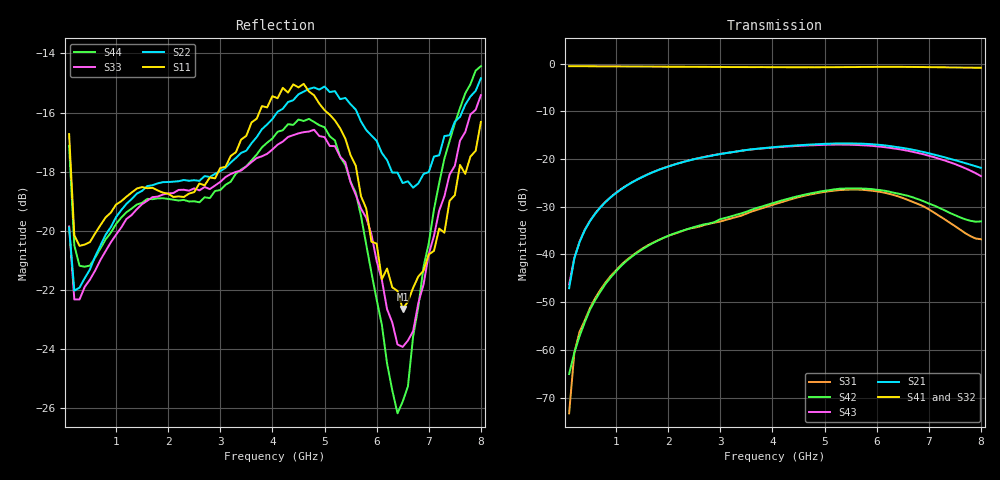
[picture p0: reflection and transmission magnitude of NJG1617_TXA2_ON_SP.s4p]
! Created Wed Nov 12 21:19:47 2008
# hz S ma R 50
! 4 Port Network Data from SP1.SP block
! freq  magS11  angS11  magS12  angS12  magS13  angS13  magS14  angS14
!  magS21  angS21  magS22  angS22  magS23  angS23  magS24  angS24
!  magS31  angS31  magS32  angS32  magS33  angS33  magS34  angS34
!  magS41  angS41  magS42  angS42  magS43  angS43  magS44  angS44
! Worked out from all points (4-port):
!   80 points, 100 MHz to 8 GHz, reference 50 ohm
!   strongest paths, dB at 100 MHz, 2.1 GHz, 4.1 GHz, 6.1 GHz, 8 GHz:
!     S41: -0.6, -0.7, -0.8, -0.7, -0.9
!     S32: -0.5, -0.7, -0.8, -0.7, -1.0
!     S21: -47.1, -21.2, -17.4, -17.1, -21.9
!     S43: -46.3, -21.2, -17.5, -17.5, -23.6
!     S42: -65.0, -35.7, -29.0, -26.6, -33.1
!     S31: -73.3, -35.7, -29.3, -27.0, -36.8
!   lowest |S11| = -22.6 dB at 6.5 GHz (marker M1), VSWR 1.16, Z = 47.3 - j6.64 ohm
!   |S11| at or under -10 dB: start of sweep to end of sweep
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1e8  0.1457 64.7  0.004651 69.8  0.0005039 148.8  0.9386 -8.5
     0.004425 77.5  0.1013 52.7  0.9429 -6.3  0.000954 106.6
     0.0002167 82.8  0.9414 -6.2  0.1017 57.0  0.004587 60.9
     0.9375 -8.4  0.0005592 95.9  0.004852 70.9  0.1391 54.1
2e8  0.09827 48.1  0.009092 80.1  0.0009035 99.5  0.9371 -6.6
     0.009065 79.9  0.07919 35.8  0.9345 -5.3  0.0009284 95.9
     0.0009352 96.7  0.9347 -5.2  0.07652 37.5  0.009224 78.7
     0.9374 -6.5  0.0009347 94.5  0.009199 79.1  0.0944 37.5
5e8  0.0957 39.3  0.02232 79.7  0.00273 102.3  0.9363 -10.2
     0.02234 79.8  0.08603 35.1  0.9348 -9.3  0.002599 102.3
     0.002744 101.9  0.9352 -9.3  0.0827 36.4  0.02252 78.8
     0.9363 -10.1  0.002642 102.8  0.02248 79.1  0.08734 34.5
1.5e9  0.1185 31.8  0.06457 66.2  0.01153 88.4  0.9286 -25.7
       0.06451 66.4  0.1168 32.5  0.9289 -24.6  0.01132 89.6
       0.01149 88.4  0.93 -24.4  0.1109 39.6  0.06491 65.2
       0.9297 -25.5  0.01129 89.8  0.06481 65.4  0.1115 36.3
5e9  0.16 -24.8  0.1442 15.4  0.04524 31.6  0.9143 -82.7
     0.1441 15.4  0.1754 -22.4  0.9127 -79.8  0.04636 30.4
     0.04528 31.8  0.9131 -79.7  0.144 17.5  0.1408 11.2
     0.9152 -82.6  0.04639 30.5  0.1408 11.3  0.1497 14.8
6.5e9  0.07374 -108.5  0.1306 -12.6  0.03904 -26.0  0.9218 -110.4
       0.1306 -12.5  0.1204 -99.1  0.9195 -106.6  0.04225 -25.9
       0.03908 -25.8  0.9196 -106.4  0.06361 50.2  0.1246 -20.0
       0.9223 -110.2  0.04233 -25.8  0.1248 -19.8  0.05142 62.7
8e9  0.1528 174.7  0.08078 -30.4  0.01442 -112.9  0.902 -140.8
     0.08077 -30.3  0.1811 179.1  0.8934 -136.6  0.02212 -113.6
     0.01443 -112.7  0.8943 -136.6  0.1696 86.6  0.06619 -58.3
     0.9023 -140.8  0.02218 -113.5  0.06625 -58.2  0.1899 85.5
